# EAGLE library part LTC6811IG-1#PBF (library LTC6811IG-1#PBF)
12 Channel Multicell Battery Monitor with Daisy Chain Interface, Generation 4 Source: Datasheet
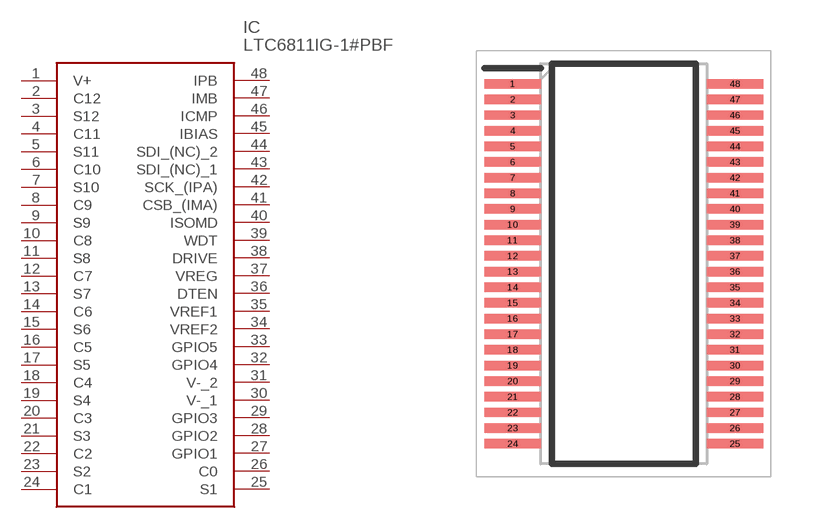
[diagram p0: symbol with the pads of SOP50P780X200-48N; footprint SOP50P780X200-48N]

Designator prefix IC

## LTC6811IG-1#PBF (Arrow_Part_Number: LTC6811IG-1#PBF; Arrow_Price-Stock: https://www.arrow.com/en/products/ltc6811ig-1pbf/analog-devices?region=nac; Description: 12 Channel Multicell Battery Monitor with Daisy Chain Interface, Generation 4; Height: 2mm; Manufacturer_Name: Analog Devices; Manufacturer_Part_Number: LTC6811IG-1#PBF)  [SOP50P780X200-48N]
1  V+
2  C12
3  S12
4  C11
5  S11
6  C10
7  S10
8  C9
9  S9
10  C8
11  S8
12  C7
13  S7
14  C6
15  S6
16  C5
17  S5
18  C4
19  S4
20  C3
21  S3
22  C2
23  S2
24  C1
25  S1
26  C0
27  GPIO1
28  GPIO2
29  GPIO3
30  V-_1
31  V-_2
32  GPIO4
33  GPIO5
34  VREF2
35  VREF1
36  DTEN
37  VREG
38  DRIVE
39  WDT
40  ISOMD
41  CSB_(IMA)
42  SCK_(IPA)
43  SDI_(NC)_1
44  SDI_(NC)_2
45  IBIAS
46  ICMP
47  IMB
48  IPB

## Footprint SOP50P780X200-48N (pad centres in mm)
SSOP 5.3 MM
smd 1.8 x 0.3: 1 -3.55,5.75; 2 -3.55,5.25; 3 -3.55,4.75; 4 -3.55,4.25; 5 -3.55,3.75; 6 -3.55,3.25; 7 -3.55,2.75; 8 -3.55,2.25; 9 -3.55,1.75; 10 -3.55,1.25; 11 -3.55,0.75; 12 -3.55,0.25; 13 -3.55,-0.25; 14 -3.55,-0.75; 15 -3.55,-1.25; 16 -3.55,-1.75; 17 -3.55,-2.25; 18 -3.55,-2.75; 19 -3.55,-3.25; 20 -3.55,-3.75; 21 -3.55,-4.25; 22 -3.55,-4.75; 23 -3.55,-5.25; 24 -3.55,-5.75; 25 3.55,-5.75; 26 3.55,-5.25; 27 3.55,-4.75; 28 3.55,-4.25; 29 3.55,-3.75; 30 3.55,-3.25; 31 3.55,-2.75; 32 3.55,-2.25; 33 3.55,-1.75; 34 3.55,-1.25; 35 3.55,-0.75; 36 3.55,-0.25; 37 3.55,0.25; 38 3.55,0.75; 39 3.55,1.25; 40 3.55,1.75; 41 3.55,2.25; 42 3.55,2.75; 43 3.55,3.25; 44 3.55,3.75; 45 3.55,4.25; 46 3.55,4.75; 47 3.55,5.25; 48 3.55,5.75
